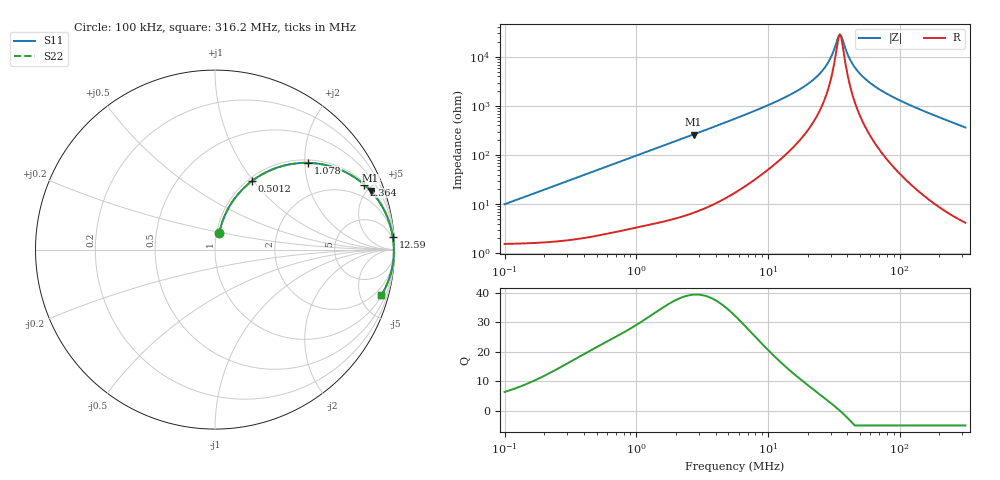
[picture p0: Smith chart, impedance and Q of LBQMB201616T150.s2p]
! LBQMB201616T150  S-PARAMETER MODEL  ( General Type )
! Model Generated by TAIYO YUDEN Corporation (http://www.ty-top.com)
! Version 1.0
! TAIYO YUDEN Control No. 191025NI43SB-FBB
! Copyright(c) 2019 TAIYO YUDEN CO.,LTD. All Rights Reserved.
! Product Description (link to TY-COMPAS)
! https://ds.yuden.co.jp/TYCOMPAS/or/detail?pn=LBQMB201616T150J&u=M
! Products Name : Inductors
! Characteristics :
!  Inductance : 15 uH , SRF(min) : 20 MHz , DC Resistance(max) : 1.95 Ohm , Rated Current : 190 mA
!  Case Size : 2.0 x 1.6 / 0.079 x 0.063 [mm/inch] , Thickness : 1.6 / 0.063 [mm/inch]
!  (Conditions: Temperature = 25 degC , DC Bias Current/Voltage = 0A / 0V)
! External Node Assignments :
!  1  o---GGG---o  2
! GND o---------o GND
! Frequency Range : 0.1MHz  -  316.199832MHz  [ 402 STEP ]
# MHz S RI R 50
! Freq[MHz].  S11 Real  S11 Imag  S21 Real  S21 Imag  S12 Real  S12 Imag  S22 Real  S22 Imag
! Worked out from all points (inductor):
!   401 points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, 100 kHz to 316.2 MHz, reference 50 ohm
!   read as one part in series: L = 15.6 uH near 104.1 kHz
!   highest Q = 39.4 at 2.723 MHz (marker M1), where L = 15.3 uH
!   self-resonance near 35.17 MHz
!   S11 on the Smith chart (normalised r, x): 100 kHz: 1.03, +0.20; 501.2 kHz: 1.05, +0.98; 1.078 MHz: 1.07, +2.08; 2.364 MHz: 1.12, +4.54; 12.59 MHz: 3, +27; 316.2 MHz: 1.08, -7.29
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0.1  0.0243 0.0943  0.9757 -0.0943  0.9757 -0.0943  0.0243 0.0943
0.219405  0.0587 0.1991  0.9413 -0.1991  0.9413 -0.1991  0.0587 0.1991
0.385695  0.1373 0.3186  0.8627 -0.3186  0.8627 -0.3186  0.1373 0.3186
0.501178  0.2036 0.3802  0.7964 -0.3802  0.7964 -0.3802  0.2036 0.3802
1.077677  0.5188 0.4833  0.4812 -0.4833  0.4812 -0.4833  0.5188 0.4833
1.487603  0.6672 0.4568  0.3328 -0.4568  0.3328 -0.4568  0.6672 0.4568
2.364476  0.8314 0.3618  0.1686 -0.3618  0.1686 -0.3618  0.8314 0.3618
2.722603  0.8664 0.3278  0.1336 -0.3278  0.1336 -0.3278  0.8664 0.3278
5.623165  0.9629 0.174  0.0371 -0.174  0.0371 -0.174  0.9629 0.174
12.58859  0.9904 0.0718  0.00965 -0.0718  0.00965 -0.0718  0.9904 0.0718
21.68824  0.9951 0.03  0.00489 -0.03  0.00489 -0.03  0.9951 0.03
28.18209  0.9961 0.0134  0.00391 -0.0134  0.00391 -0.0134  0.9961 0.0134
30.54729  0.9963 0.00854  0.00371 -0.00854  0.00371 -0.00854  0.9963 0.00854
33.78487  0.9965 0.00248  0.00353 -0.00248  0.00353 -0.00248  0.9965 0.00248
35.17403  0.9965 6.41e-05  0.00348 -6.41e-05  0.00348 -6.41e-05  0.9965 6.41e-05
36.6203  0.9966 -0.00236  0.00343 0.00236  0.00343 0.00236  0.9966 -0.00236
42.16686  0.9966 -0.0109  0.00338 0.0109  0.00338 0.0109  0.9966 -0.0109
48.5535  0.9965 -0.0198  0.00348 0.0198  0.00348 0.0198  0.9965 -0.0198
60.59956  0.996 -0.0346  0.00404 0.0346  0.00404 0.0346  0.996 -0.0346
83.65039  0.9939 -0.0595  0.00612 0.0595  0.00612 0.0595  0.9939 -0.0595
150.0428  0.9825 -0.1218  0.0175 0.1218  0.0175 0.1218  0.9825 -0.1218
316.1998  0.9274 -0.2538  0.0726 0.2538  0.0726 0.2538  0.9274 -0.2538
